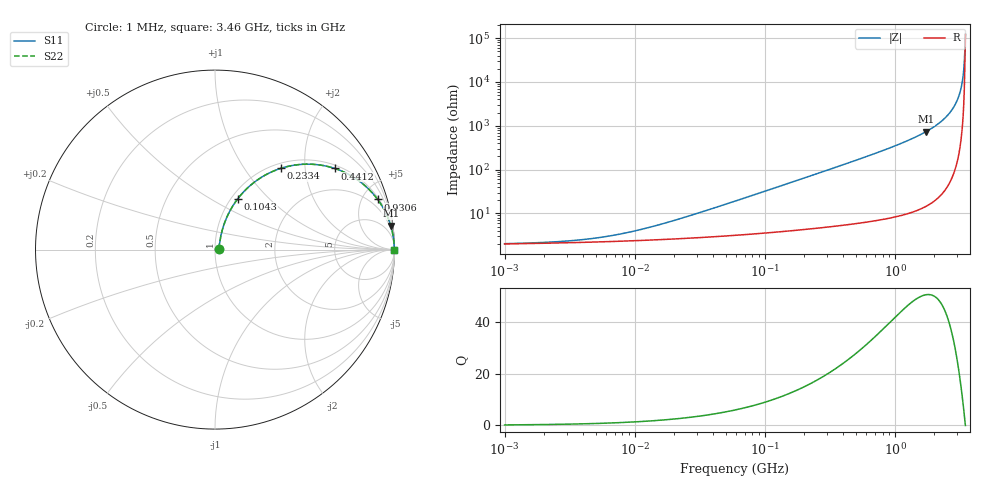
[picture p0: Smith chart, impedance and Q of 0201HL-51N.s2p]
# MHz  S  MA  R  50
!Freq  MagS11  AngS11  MagS21  AngS21  MagS12  AngS12  MagS22  AngS22
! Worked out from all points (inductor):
!   820 points, 1 MHz to 3.46 GHz, reference 50 ohm
!   read as one part in series: L = 51 nH near 25.63 MHz
!   highest Q = 50.6 at 1.725 GHz (marker M1), where L = 67.9 nH
!   self-resonance near 3.427 GHz
!   S11 on the Smith chart (normalised r, x): 1 MHz: 1.04, +0.01; 104.3 MHz: 1.07, +0.67; 233.4 MHz: 1.09, +1.50; 441.2 MHz: 1.11, +2.87; 930.6 MHz: 1.16, +6.43; 3.46 GHz: open
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1  0.02007 8.8  0.9802 -0.2  0.9802 -0.2  0.02007 8.8
3.908663  0.02469 29.1  0.9785 -0.7  0.9785 -0.7  0.02469 29.1
7.613078  0.03293 45.0  0.977 -1.4  0.977 -1.4  0.03293 45.0
15.12638  0.05323 59.8  0.9743 -2.7  0.9743 -2.7  0.05323 59.8
59.12392  0.1832 70.1  0.9533 -10.4  0.9533 -10.4  0.1832 70.1
104.2513  0.3089 65.9  0.9185 -17.9  0.9185 -17.9  0.3089 65.9
155.216  0.4335 59.8  0.8671 -25.6  0.8671 -25.6  0.4335 59.8
228.8074  0.5772 51.3  0.7823 -35.2  0.7823 -35.2  0.5772 51.3
233.4064  0.5848 50.9  0.7769 -35.7  0.7769 -35.7  0.5848 50.9
320.92  0.7036 42.6  0.6775 -44.7  0.6775 -44.7  0.7036 42.6
441.246  0.8065 34.1  0.5607 -53.7  0.5607 -53.7  0.8065 34.1
631.321  0.8917 25.2  0.4259 -63.0  0.4259 -63.0  0.8917 25.2
894.331  0.9439 17.9  0.3073 -70.7  0.3073 -70.7  0.9439 17.9
930.6444  0.9483 17.1  0.2949 -71.4  0.2949 -71.4  0.9483 17.1
1724.682  0.9883 7.7  0.1344 -81.1  0.1344 -81.1  0.9883 7.7
2395.048  0.9962 3.9  0.06759 -84.8  0.06759 -84.8  0.9962 3.9
2672.08  0.9976 2.7  0.047 -85.8  0.047 -85.8  0.9976 2.7
2922.414  0.9985 1.7  0.03054 -86.2  0.03054 -86.2  0.9985 1.7
3102.202  0.9988 1.1  0.0197 -86.0  0.0197 -86.0  0.9988 1.1
3228.163  0.999 0.7  0.01251 -85.1  0.01251 -85.1  0.999 0.7
3293.05  0.9991 0.5  0.008926 -83.8  0.008926 -83.8  0.9991 0.5
3460  0.9992 -0.0  0.0008258 2.4  0.0008258 2.4  0.9992 -0.0
